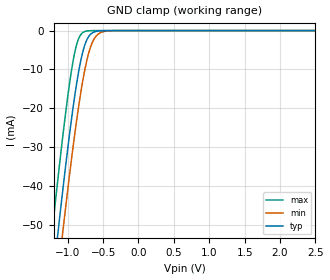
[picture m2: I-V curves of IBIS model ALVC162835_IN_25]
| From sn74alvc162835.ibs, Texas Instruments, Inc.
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[Model]   ALVC162835_IN_25
Model_type  Input
Vinl=0.7
Vinh=1.7
| variable   typ   min   max
C_comp   10.87pF   10.58pF   11.01pF
[Temperature Range]   40   100   -40
| Ambient temperature   25   85   -40
[Voltage range]   2.5   2.3   2.7
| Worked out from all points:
|   GND clamp passes 1 mA (typ) near -0.68 V on its own axis
[GND Clamp]
| ALVC162835_IN_25
|   Voltage   I(typ)   I(min)   I(max)
-2.5V     -300mA     -309.4mA   -288.3mA
-1.22V    -65.92mA   -76.78mA   -51.96mA
-1.15V    -54.2mA    -65.07mA   -40.19mA
-1.125V   -50.1mA    -60.96mA   -36.1mA
-1.07V    -41.27mA   -52.08mA   -27.39mA
-980mV    -27.63mA   -38.14mA   -14.46mA
-910mV    -18.08mA   -28.05mA   -6.523mA
-845mV    -10.58mA   -19.54mA   -2.069mA
-780mV    -5.041mA   -12.24mA   -440.8uA
-655mV    -630uA     -3.209mA   -15.41uA
-485mV    -21.18uA   -229.2uA   -148.8nA
2.5V      1.112nA    59.61nA    4.652pA
